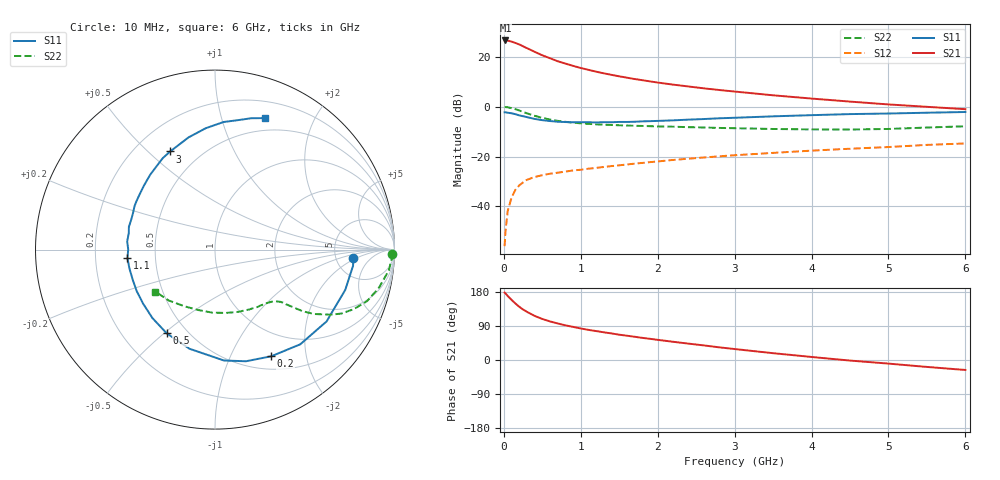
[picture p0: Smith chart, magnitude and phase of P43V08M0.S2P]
! SIEMENS Small Signal Semiconductors
! BFP182
! Si NPN RF Bipolar Junction Transistor in SOT143
! VCE = 3 V  IC = 8 mA
! Common Emitter S-Parameters:  March  1996
# GHz  S  MA  R  50
!  f  S11  S21  S12  S22
! GHz  MAG  ANG  MAG  ANG  MAG  ANG  MAG  ANG
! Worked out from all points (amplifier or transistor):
!   36 points, 10 MHz to 6 GHz, reference 50 ohm
!   highest |S21| = 26.6 dB at 20 MHz (marker M1)
!   |S21| within 3 dB of that: start of sweep to 294.6 MHz
!   unconditionally stable (mu >= 1): 1.295 GHz to 5.459 GHz
!   at 250 MHz: K = 0.29, MSG = 27.3 dB, |S12| = -30.3 dB
!   at 1.4 GHz: K = 1.04, MAG = 17.1 dB, |S12| = -23.8 dB
!   at 6 GHz: K = 0.92, MSG = 6.9 dB, |S12| = -14.7 dB
!   lowest NFmin = 1.40 dB at 450 MHz
!   S11 on the Smith chart (normalised r, x): 10 MHz: 7.41, -1.69; 200 MHz: 0.67, -1.44; 500 MHz: 0.39, -0.51; 1.1 GHz: 0.34, -0.04; 3 GHz: 0.34, +0.59; 6 GHz: 0.36, +1.39
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0.01  0.7727 -3.4  21.35 177.8  0.0016 82.3  0.9854 -1.3
0.02  0.7744 -6.7  21.36 176.0  0.003 84.0  0.9872 -2.7
0.05  0.7596 -17.2  21.2 169.0  0.0081 81.8  0.9754 -6.8
0.1  0.7393 -32.8  20.25 158.7  0.015 72.4  0.9379 -13.1
0.15  0.71 -48.0  19.03 149.2  0.0216 66.6  0.8948 -18.7
0.2  0.6719 -62.2  17.79 140.5  0.0265 61.8  0.8417 -23.2
0.25  0.6456 -74.5  16.29 133.2  0.0304 56.5  0.7881 -26.9
0.3  0.6199 -85.4  14.98 127.2  0.0343 53.0  0.7388 -29.4
0.4  0.5705 -104.4  12.66 116.4  0.039 47.9  0.6588 -33.0
0.5  0.5384 -120.0  10.76 108.3  0.0425 44.3  0.5978 -35.1
0.6  0.5168 -132.4  9.396 101.8  0.0454 42.3  0.5539 -36.1
0.7  0.5012 -143.0  8.182 96.4  0.0476 41.8  0.5219 -36.9
0.9  0.4883 -159.7  6.613 87.4  0.0528 40.9  0.4793 -38.0
1.1  0.4902 -174.4  5.5 79.5  0.0573 41.0  0.4536 -39.6
1.5  0.4962 165.2  4.076 66.8  0.067 41.3  0.4251 -43.4
1.8  0.5095 151.7  3.412 58.4  0.0748 41.3  0.412 -47.2
2.2  0.5335 137.7  2.779 48.1  0.0857 40.3  0.3982 -53.4
3  0.6012 114.5  2.02 28.9  0.1066 36.4  0.3714 -68.8
3.5  0.6422 103.3  1.697 18.0  0.1188 33.3  0.3582 -80.1
4.5  0.7124 86.2  1.269 -1.5  0.144 26.7  0.3496 -105.8
5.5  0.7591 74.6  0.997 -18.3  0.172 19.9  0.383 -132.2
6  0.7848 69.0  0.894 -26.3  0.1837 15.3  0.4062 -144.8
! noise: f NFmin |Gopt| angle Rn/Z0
0.45  1.4  0.26  41  0.29
0.9  1.5  0.25  83  0.23
1.8  2  0.21  162  0.2
